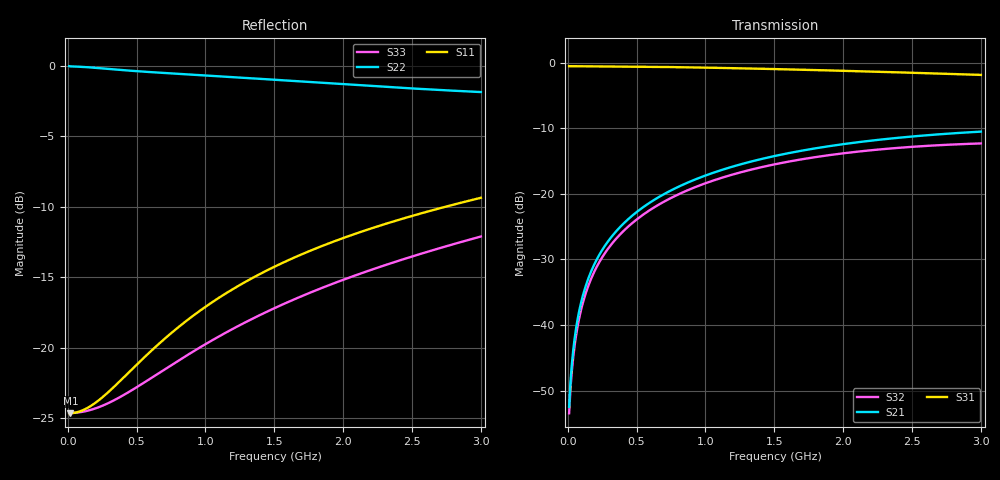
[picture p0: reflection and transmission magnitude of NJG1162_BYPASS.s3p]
! Created Tue Oct 27 16:08:58 2020
# hz S ma R 50
! 3 Port Network Data from SP1.SP block
! freq  magS11  angS11  magS12  angS12  magS13  angS13
!  magS21  angS21
!  magS22  angS22  magS23  angS23
!  magS31  angS31  magS32  angS32
!  magS33  angS33
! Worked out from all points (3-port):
!   300 points, 10 MHz to 3 GHz, reference 50 ohm
!   strongest paths, dB at 10 MHz, 760 MHz, 1.51 GHz, 2.26 GHz, 3 GHz:
!     S31: -0.5, -0.7, -1.0, -1.4, -1.9
!     S21: -52.5, -19.4, -14.2, -11.8, -10.5
!     S32: -53.4, -20.5, -15.5, -13.2, -12.3
!   lowest |S11| = -24.7 dB at 20 MHz (marker M1), VSWR 1.12, Z = 56.2 - j0.373 ohm
!   |S11| at or under -10 dB: start of sweep to 2.747 GHz
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1e7  0.05853 -1.7  0.002362 61.9  0.9388 -0.2
     0.002374 62.5  0.9954 -0.6  0.002139 63.8
     0.9388 -0.2  0.002127 63.2  0.05875 -1.3
2e7  0.05848 -3.2  0.003656 66.4  0.9386 -0.4
     0.003704 67.1  0.9938 -1.0  0.003351 67.7
     0.9386 -0.4  0.003308 67.1  0.05867 -2.4
6e7  0.05887 -9.3  0.00916 77.7  0.9383 -1.1
     0.009365 78.1  0.992 -2.6  0.00846 78.3
     0.9383 -1.1  0.008278 77.9  0.05878 -7.0
1.2e8  0.0603 -18.2  0.01785 80.1  0.9378 -2.2
       0.01827 80.3  0.9886 -5.1  0.01648 80.5
       0.9378 -2.2  0.0161 80.3  0.05937 -13.7
2.2e8  0.06475 -31.7  0.03218 78.6  0.9365 -3.9
       0.03297 78.7  0.9803 -9.1  0.02969 79.2
       0.9365 -3.9  0.02899 79.1  0.06133 -24.4
3.6e8  0.0745 -47.4  0.05175 74.9  0.9342 -6.4
       0.05303 75.0  0.9673 -14.3  0.04771 75.8
       0.9342 -6.4  0.04658 75.8  0.06597 -38.1
8.1e8  0.1188 -79.1  0.1112 61.5  0.9221 -14.1
       0.114 61.6  0.9346 -29.7  0.1023 63.5
       0.9221 -14.1  0.09977 63.5  0.0903 -71.5
1.51e9  0.1945 -105.4  0.19 40.5  0.8918 -25.7
        0.1949 40.5  0.8903 -52.3  0.1727 44.0
        0.8919 -25.7  0.1684 44.1  0.1386 -104.0
2.2e9  0.2643 -122.8  0.2474 20.8  0.854 -36.6
       0.254 20.8  0.8469 -72.7  0.2204 25.9
       0.8541 -36.7  0.2147 26.1  0.1885 -126.4
3e9  0.3399 -138.9  0.2897 -0.5  0.8053 -49.0
     0.2978 -0.5  0.8058 -93.8  0.2491 6.5
     0.8054 -49.0  0.2421 6.8  0.2478 -147.3
